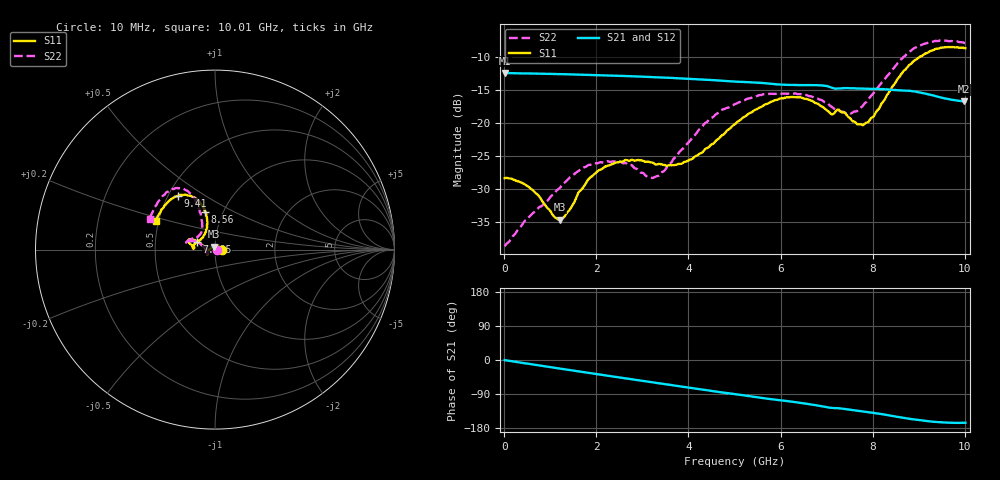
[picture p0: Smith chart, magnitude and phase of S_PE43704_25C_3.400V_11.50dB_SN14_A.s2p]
! Device ID: PE43704
! Dir: z:\PE43704\PE43704_Char_1_20130516\PE43704\AMB\3p400V\11p50dB
! Serial: 14
! Insertion: A
! Impedance: 50 ohm
! Temp: Amb
! VDD: 3.400V
! Attenuation Step: 11.50dB
! IDD: 1.139731e-01mA
#  Hz  S  RI  R  50
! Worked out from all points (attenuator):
!   401 points, 10 MHz to 10.01 GHz, reference 50 ohm
!   highest |S21| = -12.48 dB at 10 MHz (marker M1); lowest = -16.8 dB at 9.985 GHz (marker M2)
!   lowest |S11| = -34.7 dB at 1.21 GHz (marker M3), VSWR 1.04, Z = 49.1 + j1.62 ohm
!   |S11| at or under -10 dB: start of sweep to 9.029 GHz
!   |S22| runs from -38.6 to -7.6 dB; largest |S21 - S12| = 0.0018
!   S11 on the Smith chart (normalised r, x): 10 MHz: 1.08, +0.00; 7.485 GHz: 0.81, +0.07; 8.56 GHz: 0.82, +0.37; 9.41 GHz: 0.56, +0.39; 10.01 GHz: 0.48, +0.18
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1e7  0.0382 0.000281  0.2376 -0.000871  0.2376 -0.000846  0.0117 0.000373
5.1e8  0.028 0.0179  0.2324 -0.0396  0.2323 -0.0396  0.00354 0.0185
1.21e9  -0.00835 0.0165  0.2151 -0.0897  0.2151 -0.0897  -0.0281 0.0158
1.685e9  -0.0316 -0.000445  0.1971 -0.12  0.1972 -0.12  -0.0453 -0.00222
2.01e9  -0.0405 -0.0127  0.1823 -0.1386  0.1824 -0.1385  -0.0474 -0.0138
2.41e9  -0.0437 -0.0239  0.1618 -0.1589  0.1618 -0.1588  -0.0464 -0.0207
3.16e9  -0.0421 -0.0276  0.1177 -0.1877  0.1179 -0.1878  -0.0372 -0.00998
3.36e9  -0.0429 -0.0235  0.1051 -0.1934  0.1052 -0.1932  -0.0397 -0.00333
4.06e9  -0.0528 0.000836  0.0597 -0.2057  0.06 -0.2056  -0.0713 0.0237
4.46e9  -0.0641 0.0174  0.0335 -0.2083  0.0337 -0.2085  -0.0974 0.0441
5.01e9  -0.0893 0.0394  -0.000255 -0.2045  -6.3e-05 -0.2046  -0.1301 0.0466
5.96e9  -0.1392 0.0578  -0.0528 -0.1876  -0.0521 -0.1875  -0.1587 0.046
6.685e9  -0.1422 0.0347  -0.0897 -0.1701  -0.0897 -0.17  -0.1494 0.049
7.185e9  -0.1203 0.00533  -0.1088 -0.1443  -0.1086 -0.1451  -0.1095 0.0618
7.485e9  -0.102 0.0404  -0.1194 -0.1378  -0.1193 -0.138  -0.0876 0.0812
7.86e9  -0.0639 0.0771  -0.1319 -0.1235  -0.132 -0.1238  -0.0721 0.124
8.36e9  -0.0438 0.1658  -0.1479 -0.0986  -0.1475 -0.0993  -0.0858 0.2192
8.56e9  -0.0542 0.2119  -0.1533 -0.0865  -0.1529 -0.0867  -0.1052 0.2662
8.935e9  -0.1024 0.281  -0.1587 -0.0658  -0.1579 -0.0646  -0.164 0.3319
9.41e9  -0.205 0.2987  -0.1513 -0.0437  -0.151 -0.0436  -0.2554 0.3261
9.985e9  -0.3244 0.1691  -0.1405 -0.0357  -0.1411 -0.0358  -0.3585 0.1783
1.001e10  -0.3297 0.1593  -0.1405 -0.036  -0.1414 -0.0365  -0.3625 0.1701
